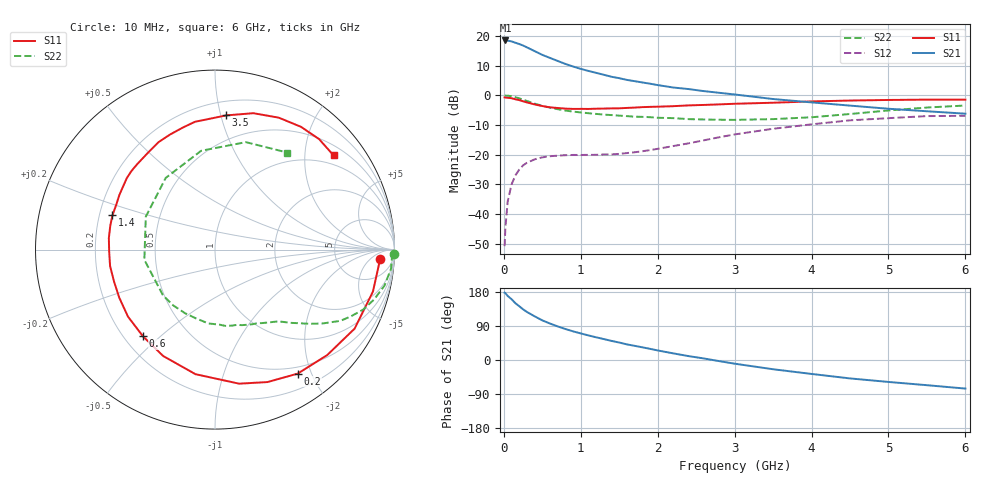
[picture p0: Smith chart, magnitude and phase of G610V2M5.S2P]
! SIEMENS Small Signal Semiconductors
! BFG193
! Si NPN RF Bipolar Junction Transistor in SOT223
! VCE = 10 V  IC = 2.5 mA
! Common Emitter S-Parameters:  August  1996
# GHz  S  MA  R  50
!  f  S11  S21  S12  S22
! GHz  MAG  ANG  MAG  ANG  MAG  ANG  MAG  ANG
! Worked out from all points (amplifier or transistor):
!   36 points, 10 MHz to 6 GHz, reference 50 ohm
!   highest |S21| = 18.5 dB at 20 MHz (marker M1)
!   |S21| within 3 dB of that: start of sweep to 353.6 MHz
!   unconditionally stable (mu >= 1): 1.342 GHz to 2.523 GHz
!   at 250 MHz: K = 0.20, MSG = 20.2 dB, |S12| = -23.6 dB
!   at 1.4 GHz: K = 1.05, MAG = 11.8 dB, |S12| = -19.9 dB
!   at 6 GHz: K = 0.92, MSG = 0.4 dB, |S12| = -6.9 dB
!   S11 on the Smith chart (normalised r, x): 10 MHz: 17, -11; 200 MHz: 0.40, -1.80; 600 MHz: 0.28, -0.44; 1.4 GHz: 0.25, +0.15; 3.5 GHz: 0.30, +1.04; 6 GHz: 0.74, +2.68
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0.01  0.9214 -3.1  8.348 177.6  0.0029 91.7  0.9952 -1.3
0.02  0.9152 -6.3  8.368 176.5  0.0059 87.3  0.9867 -2.5
0.05  0.9105 -14.9  8.286 169.0  0.0164 80.7  0.9866 -6.2
0.1  0.8939 -29.5  8.073 160.4  0.0316 74.9  0.9655 -12.0
0.15  0.8581 -43.2  7.659 149.9  0.045 66.0  0.9282 -17.5
0.2  0.8305 -56.3  7.287 142.0  0.0563 59.9  0.89 -22.1
0.25  0.7938 -68.4  6.881 133.8  0.0663 53.8  0.8432 -26.2
0.3  0.759 -79.8  6.404 126.8  0.0733 49.4  0.8036 -29.6
0.4  0.7026 -98.9  5.538 115.3  0.0837 41.2  0.7253 -34.6
0.5  0.6594 -116.0  4.788 104.6  0.0904 35.1  0.6653 -38.4
0.6  0.628 -129.7  4.251 96.2  0.0945 31.3  0.6201 -41.4
0.7  0.612 -142.4  3.785 88.6  0.0966 28.5  0.5842 -44.3
0.8  0.5969 -153.3  3.371 81.8  0.0983 26.2  0.5535 -46.7
1.1  0.5897 -178.8  2.57 64.9  0.0996 24.5  0.4995 -54.5
1.4  0.6023 161.5  2.051 50.4  0.1012 26.5  0.465 -63.4
1.6  0.6135 150.3  1.815 41.2  0.1068 29.2  0.4467 -70.4
2.2  0.656 124.8  1.354 17.6  0.1399 34.8  0.4131 -95.1
2.8  0.7036 104.6  1.102 -3.0  0.1971 31.5  0.3883 -126.8
3.5  0.7504 85.2  0.866 -24.4  0.2737 17.7  0.3977 -171.8
4.5  0.8164 64.2  0.671 -48.6  0.3792 -5.5  0.4847 124.5
5.5  0.8457 46.7  0.539 -66.5  0.4469 -34.2  0.6228 74.0
6  0.8437 38.5  0.491 -75.4  0.4522 -49.9  0.6737 53.4
